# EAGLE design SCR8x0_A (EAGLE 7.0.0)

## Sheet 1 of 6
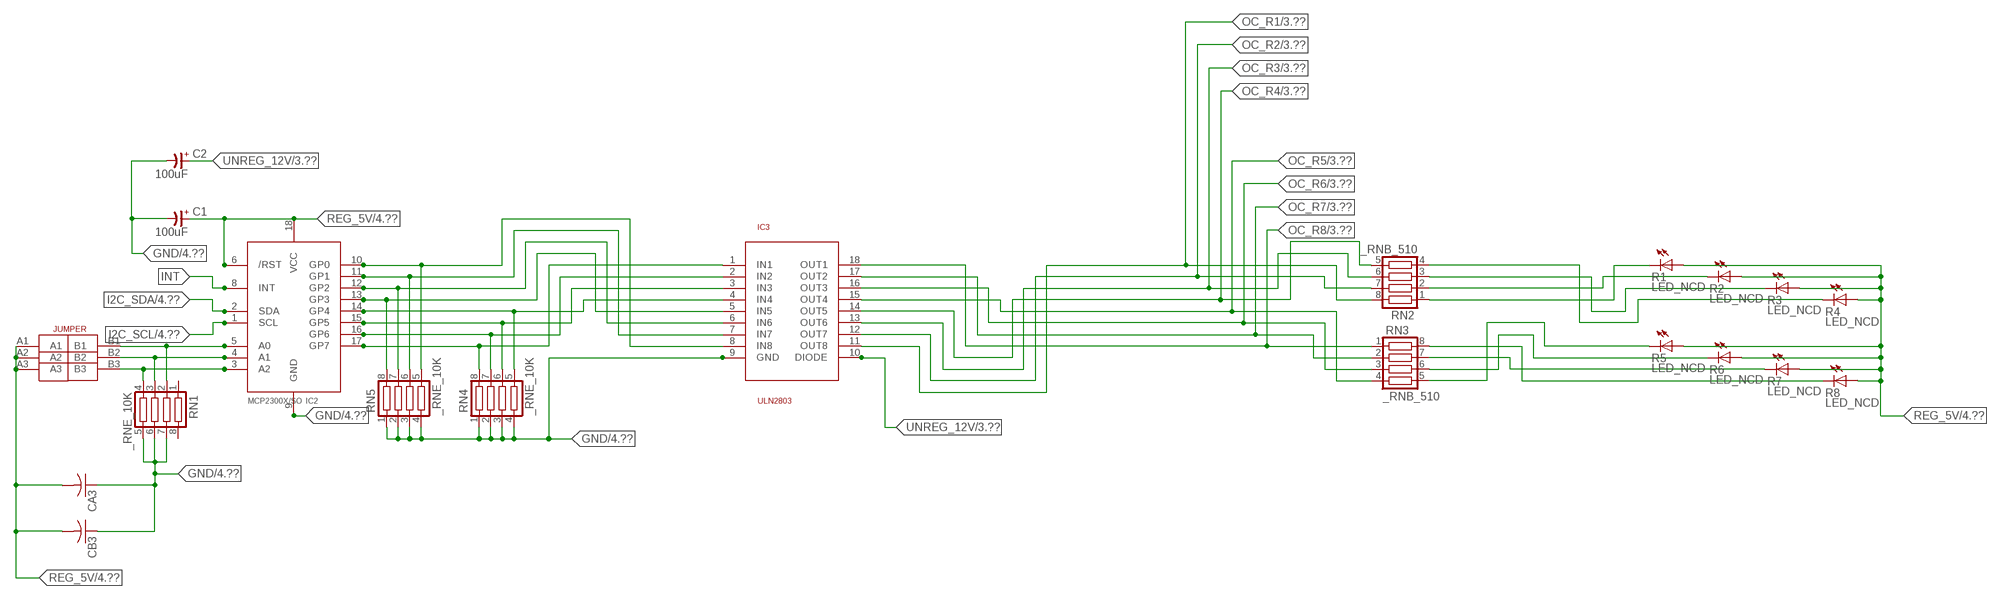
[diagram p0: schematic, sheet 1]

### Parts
C1  100uF  CP-E-025X060  [E-025X060]
C2  100uF  CP-E-025X060  [E-025X060]
CA3  CC1206KRX7R9BB104C1206K  [CC1206KRX7R9BB104]
CB3  TMK316F106ZL-TC1206K  [TMK316F106ZL-T]
IC2  MCP2300X/SO  [SO18W]
IC3  ULN2803  [SO18L]
R1  LED_NCD  [CHIPLED_0603]
R2  LED_NCD  [CHIPLED_0603]
R3  LED_NCD  [CHIPLED_0603]
R4  LED_NCD  [CHIPLED_0603]
R5  LED_NCD  [CHIPLED_0603]
R6  LED_NCD  [CHIPLED_0603]
R7  LED_NCD  [CHIPLED_0603]
R8  LED_NCD  [CHIPLED_0603]
RN1  _RNE_10K  [RNE]
RN2  _RNB_510  [RNB]
RN3  _RNB_510  [RNB]
RN4  _RNE_10K  [RNE]
RN5  _RNE_10K  [RNE]
U$18  JUMPER_3X2  [JUMPER_3X2]

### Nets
GND: C1.- C2.- CA3.1 CB3.1 IC2.9(GND) IC3.9(GND) RN1.5 RN1.6 RN1.7 RN4.1 RN4.2 RN4.3 RN4.4 RN5.1 RN5.2 RN5.3 RN5.4 ; also sheet 4,6
GP4: IC2.14(GP4) IC3.4(IN4) RN4.5
GP6: IC2.16(GP6) IC3.2(IN2) RN4.7
I2C_SCL: IC2.1(SCL) ; also sheet 4
I2C_SDA: IC2.2(SDA) ; also sheet 4
INT: IC2.8(INT)
N$6: IC2.5(A0) RN1.2 U$18.B1
N$7: IC2.4(A1) RN1.3 U$18.B2
N$8: IC2.3(A2) RN1.4 U$18.B3
N$20: R1.C RN2.1
N$21: IC2.12(GP2) IC3.6(IN6) RN5.7
N$22: IC2.11(GP1) IC3.7(IN7) RN5.6
N$23: IC2.10(GP0) IC3.8(IN8) RN5.5
N$29: R2.C RN2.2
N$30: R3.C RN2.3
N$31: R4.C RN2.4
N$32: R8.C RN3.8
N$81: R7.C RN3.7
N$82: R6.C RN3.6
N$83: R5.C RN3.5
N$89: IC2.13(GP3) IC3.5(IN5) RN5.8
N$93: IC2.15(GP5) IC3.3(IN3) RN4.6
N$94: IC2.17(GP7) IC3.1(IN1) RN4.8
OC_R1: IC3.11(OUT8) RN2.8 ; also sheet 3
OC_R2: IC3.12(OUT7) RN2.7 ; also sheet 3
OC_R3: IC3.13(OUT6) RN2.6 ; also sheet 3
OC_R4: IC3.14(OUT5) RN2.5 ; also sheet 3
OC_R5: IC3.15(OUT4) RN3.4 ; also sheet 3
OC_R6: IC3.16(OUT3) RN3.3 ; also sheet 3
OC_R7: IC3.17(OUT2) RN3.2 ; also sheet 3
OC_R8: IC3.18(OUT1) RN3.1 ; also sheet 3
REG_5V: C1.+ CA3.2 CB3.2 IC2.6(/RST) IC2.18(VCC) R1.A R2.A R3.A R4.A R5.A R6.A R7.A R8.A U$18.A1 U$18.A2 U$18.A3 ; also sheet 4,6
UNREG_12V: C2.+ IC3.10(DIODE) ; also sheet 3,4
Unconnected: RN1.1 RN1.8

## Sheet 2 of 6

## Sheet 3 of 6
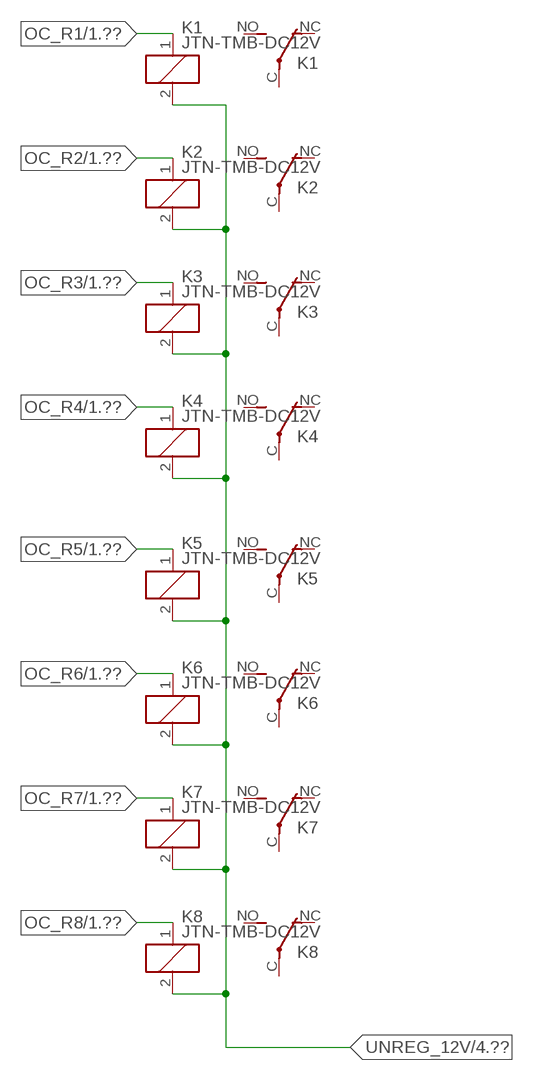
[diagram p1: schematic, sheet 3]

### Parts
K1  JTN-TMB-DC12V  [JT-TMB]
K2  JTN-TMB-DC12V  [JT-TMB]
K3  JTN-TMB-DC12V  [JT-TMB]
K4  JTN-TMB-DC12V  [JT-TMB]
K5  JTN-TMB-DC12V  [JT-TMB]
K6  JTN-TMB-DC12V  [JT-TMB]
K7  JTN-TMB-DC12V  [JT-TMB]
K8  JTN-TMB-DC12V  [JT-TMB]

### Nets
OC_R1: K1.1(C1) ; also sheet 1
OC_R2: K2.1(C1) ; also sheet 1
OC_R3: K3.1(C1) ; also sheet 1
OC_R4: K4.1(C1) ; also sheet 1
OC_R5: K5.1(C1) ; also sheet 1
OC_R6: K6.1(C1) ; also sheet 1
OC_R7: K7.1(C1) ; also sheet 1
OC_R8: K8.1(C1) ; also sheet 1
UNREG_12V: K1.2(C2) K2.2(C2) K3.2(C2) K4.2(C2) K5.2(C2) K6.2(C2) K7.2(C2) K8.2(C2) ; also sheet 1,4
Unconnected: K1.C(COM) K1.NC K1.NO K2.C(COM) K2.NC K2.NO K3.C(COM) K3.NC K3.NO K4.C(COM) K4.NC K4.NO K5.C(COM) K5.NC K5.NO K6.C(COM) K6.NC K6.NO K7.C(COM) K7.NC K7.NO K8.C(COM) K8.NC K8.NO

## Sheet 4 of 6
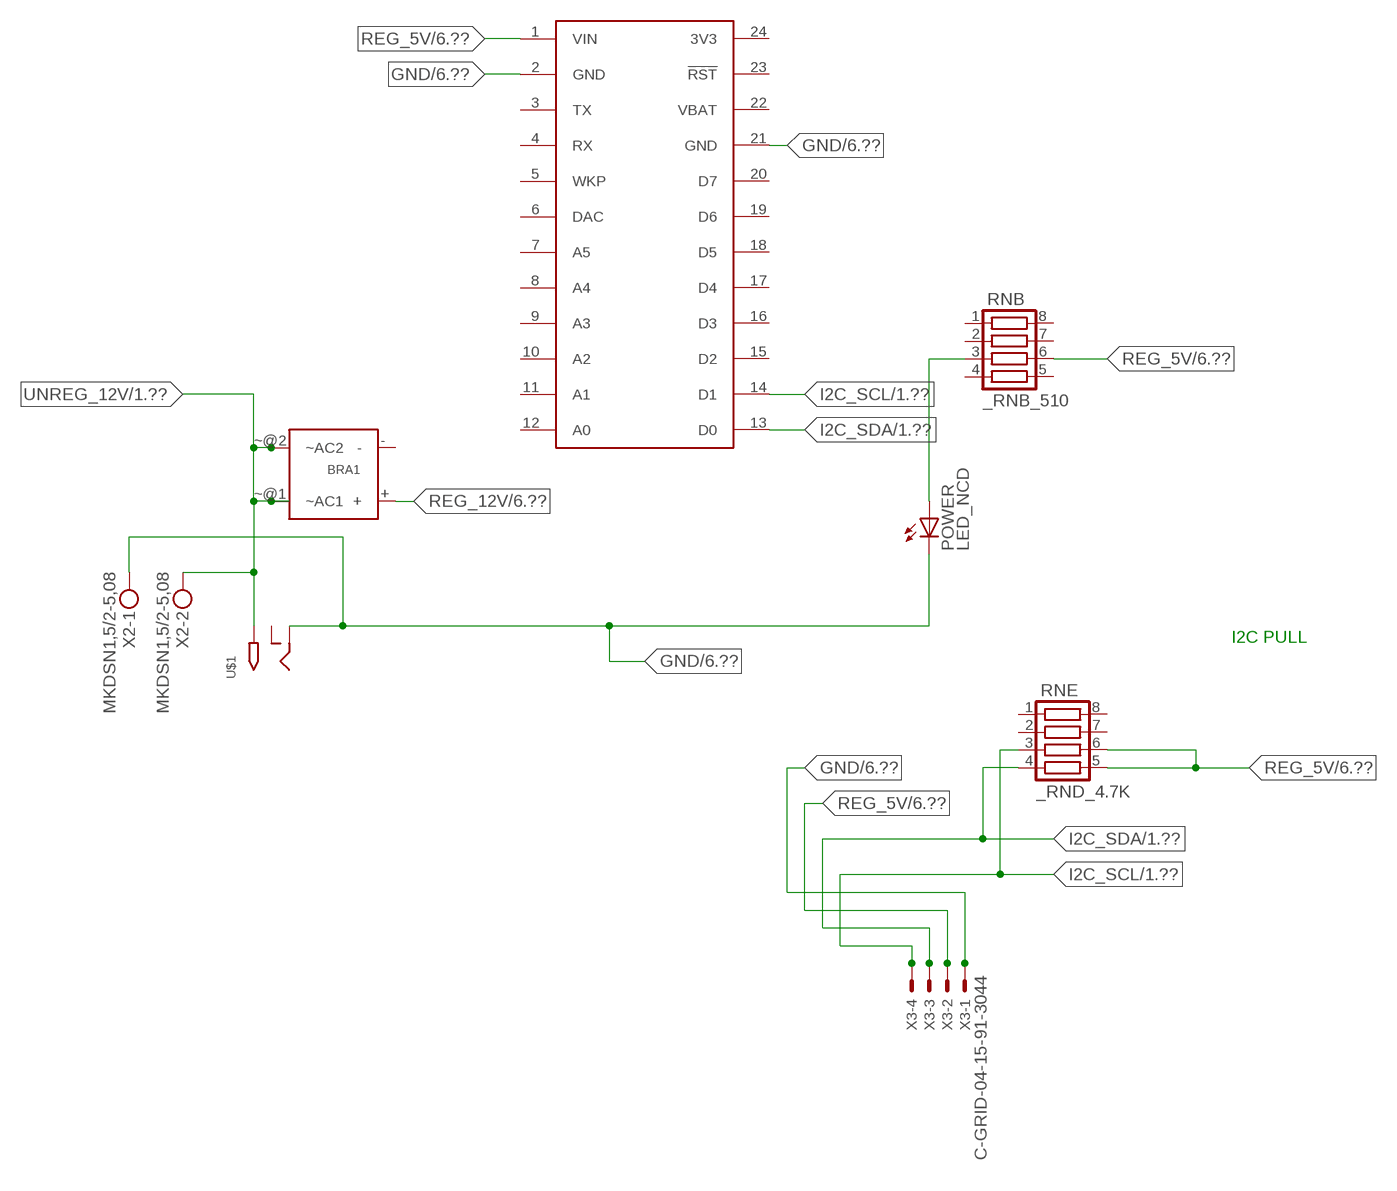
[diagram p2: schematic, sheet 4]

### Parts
BRA1  MB2S_  [MB2S]
POWER  LED_NCD  [CHIPLED_0603]
RNB  _RNB_510  [RNB]
RNE  _RND_4.7K  [RND]
S1  SPARK_CORECORE  [SPARK_CORE]
U$1  2.1MMJACK  [PJ-102A]
X2  MKDSN1,5/2-5,08  [MKDSN1,5/2-5,08]
X3  C-GRID-04-15-91-3044  [15-91-04]

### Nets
GND: POWER.C S1.2(GND) S1.21(GND) U$1.RING X2.1 X3.1 ; also sheet 1,6
I2C_SCL: RNE.3 S1.14(D1) X3.4 ; also sheet 1
I2C_SDA: RNE.4 S1.13(D0) X3.3 ; also sheet 1
N$2: POWER.A RNB.3
REG_5V: RNB.6 RNE.5 RNE.6 S1.1(VIN) X3.2 ; also sheet 1,6
REG_12V: BRA1.+ ; also sheet 6
UNREG_12V: BRA1.~@1(~AC1) BRA1.~@2(~AC2) U$1.TIP X2.2 ; also sheet 1,3
Unconnected: BRA1.- RNB.1 RNB.2 RNB.4 RNB.5 RNB.7 RNB.8 RNE.1 RNE.2 RNE.7 RNE.8 S1.3(TX) S1.4(RX) S1.5(WKP) S1.6(DAC) S1.7(A5) S1.8(A4) S1.9(A3) S1.10(A2) S1.11(A1) S1.12(A0) S1.15(D2) S1.16(D3) S1.17(D4) S1.18(D5) S1.19(D6) S1.20(D7) S1.23(!RST) U$1.RING_SW

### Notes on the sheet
- I2C PULL

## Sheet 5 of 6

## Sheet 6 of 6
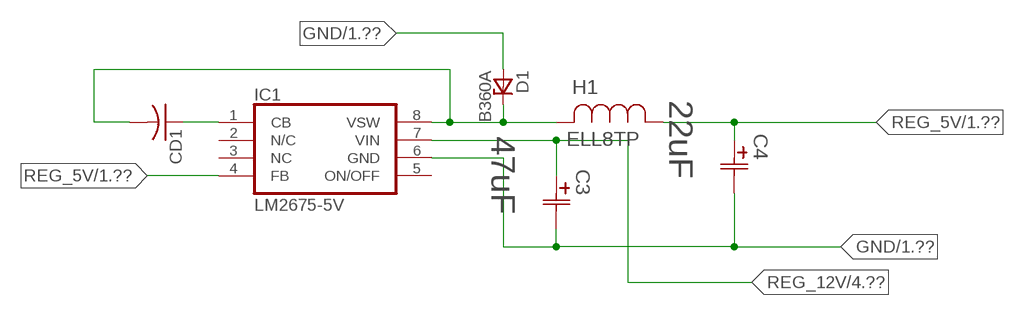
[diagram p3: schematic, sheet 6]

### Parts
C3  47uF  490-5463-6-NDCAP  [C2917(7343)-Y]
C4  22uF  490-5463-6-NDCAP  [C2917(7343)-Y]
CD1  _CD_10NF_50VC1206K  [_CD_10NF_50V]
D1  B360A  [DO214AC_ZENER]
H1  ELL8TP  [IND_ELL8TP]
IC1  LM2675-5V  LM2675  [SO-8]

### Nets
GND: C3.2(C2) C4.2(C2) D1.A IC1.6(GND) ; also sheet 1,4
N$1: CD1.2 D1.C H1.2 IC1.8(VSW)
N$3: CD1.1 IC1.1(CB)
REG_5V: C4.1(C1) H1.1 IC1.4(FB) ; also sheet 1,4
REG_12V: C3.1(C1) IC1.7(VIN) ; also sheet 4
Unconnected: IC1.2(N/C) IC1.5(ON/OFF)

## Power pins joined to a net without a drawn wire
3V3: S1.24(3V3)
NC: IC1.3(NC)
VBAT: S1.22(VBAT)

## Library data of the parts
BRA1 = NCD_ULTIMATE_LIBRARY:MB2S: Bridge Rectifier BRA MB2S 200V 500ma Digikey MB2S-TPMSTR-ND/MB2S-TP
C1 C2 = NCD_ULTIMATE_LIBRARY:CP-: Capacitors All Kinds POLARIZED CAP
C3 C4 = NCD_ULTIMATE_bhaskar:490-5463-6-ND: NCD CAP
CA3 = NCD_ULTIMATE_LIBRARY:CC1206KRX7R9BB104: Capacitor CA .1uF 50V SMT C1206K CC1206KRX7R9BB104
CB3 = NCD_ULTIMATE_LIBRARY:TMK316F106ZL-T: Capacitor CB 10uF SMT 1206 TMK316F106ZL-T
CD1 = NCD_ULTIMATE_LIBRARY:_CD_10NF_50V: Capacitor 10nF SMT
D1 = NCD_ULTIMATE_bhaskar:B360A: NCD DIODE B350A/B360A
H1 = NCD_ULTIMATE_bhaskar:ELL8TP: NCD coil
IC1 = NCD_ULTIMATE_bhaskar:LM2675: LM2675 NCD http://www.ti.com/lit/ds/symlink/lm2675.pdf
IC2 = NCD_ULTIMATE_LIBRARY:MCP2300X: Semiconductor Port Expander I/O 8-Bit I2C MCP23008 Inexpensive i2c i/o expander - 8 general purpose i/o pins with optional pullups
IC3 = NCD_ULTIMATE_LIBRARY:ULN2803: Semiconductor 8 O.C. N-Channel Transistor Driver Digikey ULN2803AFWGCELTR-ND/ULN2803AFWG,C,EL
K1-K8 = NCD_ULTIMATE_LIBRARY:JT?-*: RELAY COMPACT ECONOMICAL 30 AMP. RELAY NAiS Source: http://www.mew-europe.com/.. en_ds_61212_0000.pdf
POWER = NCD_ULTIMATE_bhaskar:LED_NCD
R1-R8 = NCD_ULTIMATE_LIBRARY:LED_NCD: LED Digikey 754-1132-2-ND/APT2012SRCPRV
RN1 RN4 RN5 = NCD_ULTIMATE_LIBRARY:_RNE_10K: Resistor Array RNE SMT 10K x 4 Single Resistor Source: http://www.ctscorp.com/components/Datasheets/CTSChipArrayDs.pdf Digikey 742C083103JPTR-ND/742C083103JP; OC_FARNELL: unknown; OC_NEWARK: unknown
RN2 RN3 RNB = NCD_ULTIMATE_LIBRARY:_RNB_510: Resistor Array RNB SMT 510 x 4 Single Resistor Source: http://www.ctscorp.com/components/Datasheets/CTSChipArrayDs.pdf Digikey 742C083511JPTR-ND/ 742C083511JP; OC_FARNELL: unknown; OC_NEWARK: unknown
RNE = NCD_ULTIMATE_LIBRARY:_RND_4.7K: Resistor Array RND SMT 4.7K x 4 Single Resistor Source: http://www.ctscorp.com/components/Datasheets/CTSChipArrayDs.pdf Digikey 742C083472JPTR-ND/742C083472JP; OC_FARNELL: unknown; OC_NEWARK: unknown
S1 = Spark:SPARK_CORE
U$1 = NCD_ULTIMATE_CONNECTORS:2.1MMJACK: 2.1mm x 5.5mm DC jack with internal switch. Digikey part #PJ-102A, 4UCON part #05537 By microbuilder.eu
U$18 = NCD_ULTIMATE_CONNECTORS:JUMPER_3X2
X2 = NCD_ULTIMATE_CONNECTORS:MKDSN1,5/2-5,08: MKDSN 1,5/ 2-5,08 Printklemme
X3 = NCD_ULTIMATE_CONNECTORS:C-GRID-04: CONNECTOR 4-Pos I2C wire to board 2.54 mm (0.100") pitch header Digikey WM1342-ND/0015912045; OC_FARNELL: unknown; OC_NEWARK: unknown

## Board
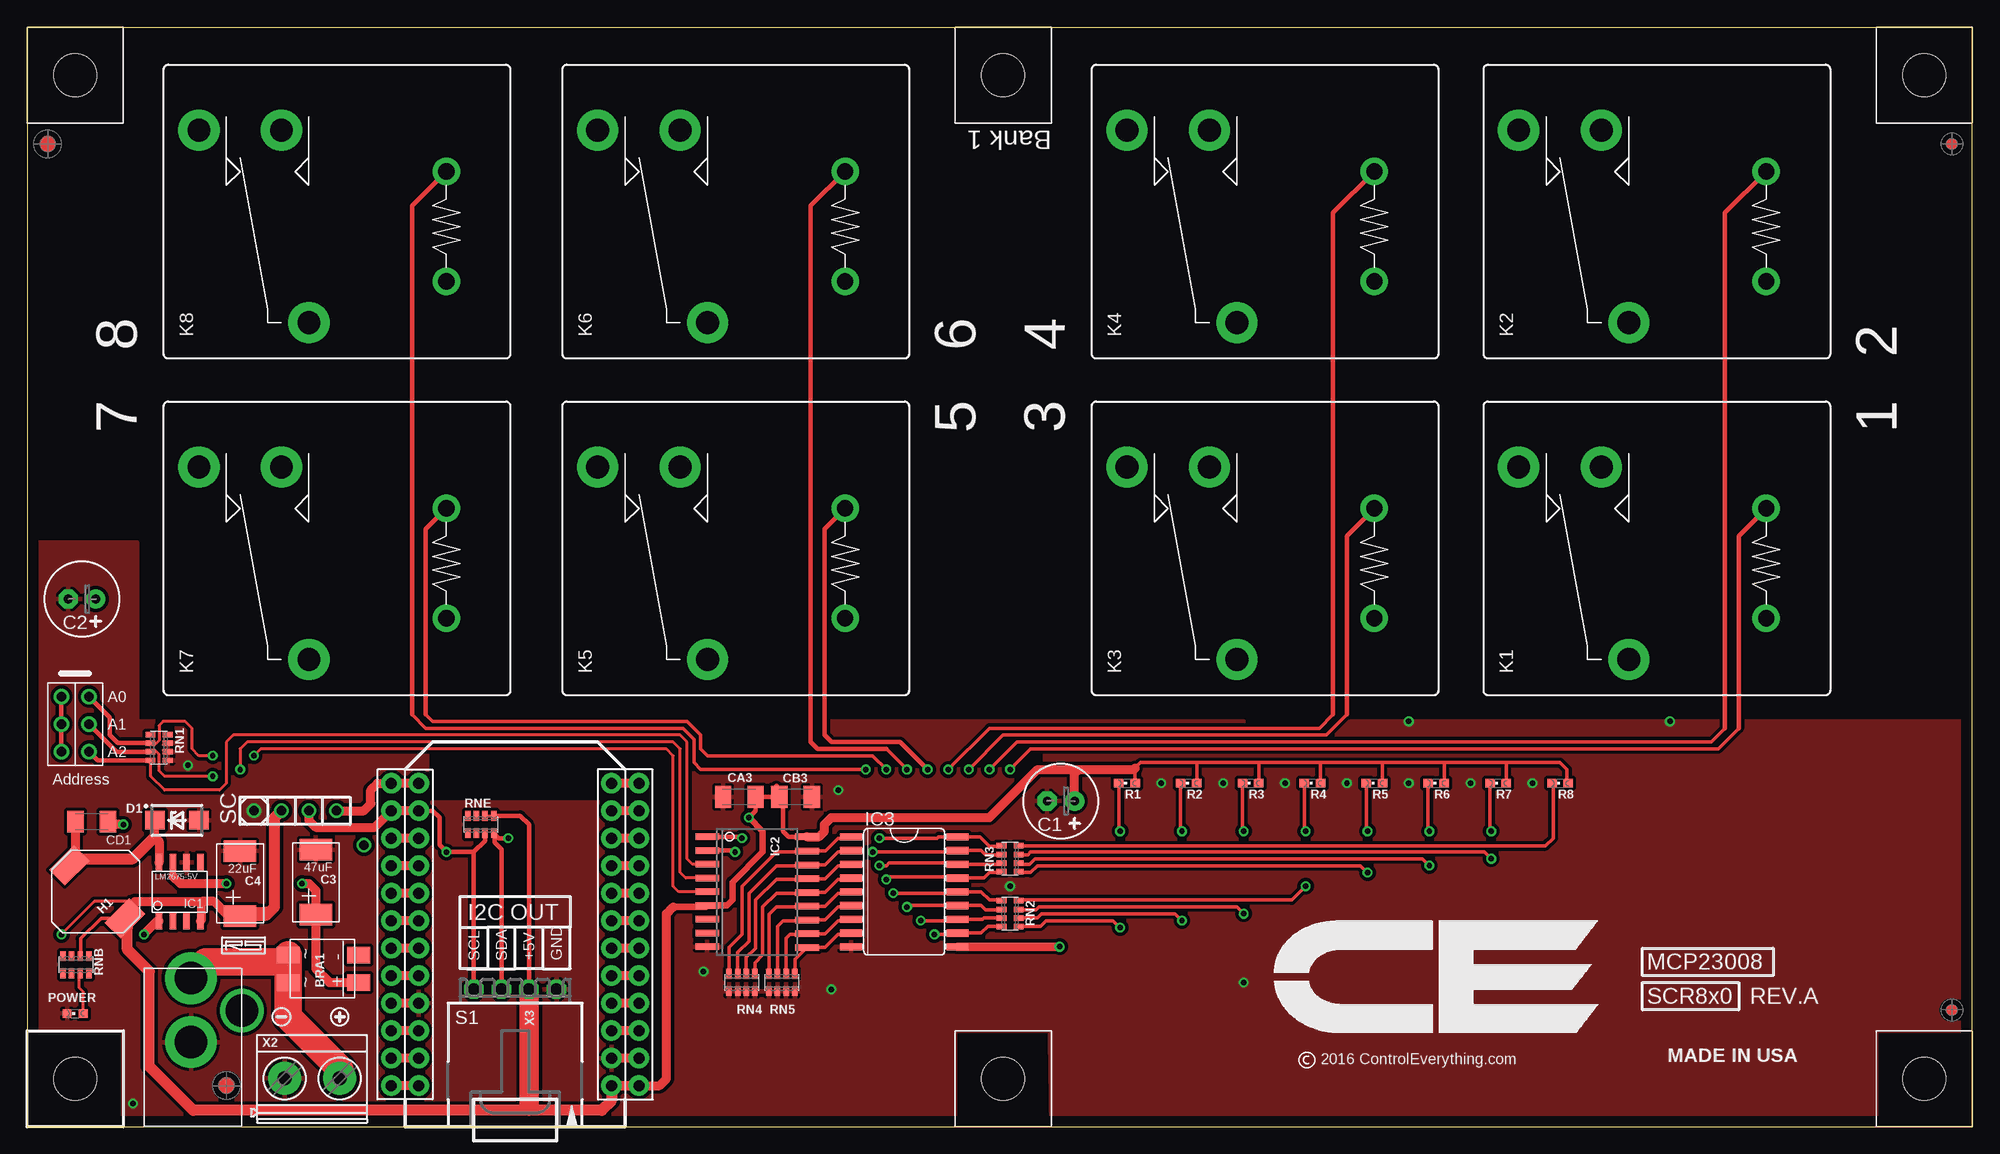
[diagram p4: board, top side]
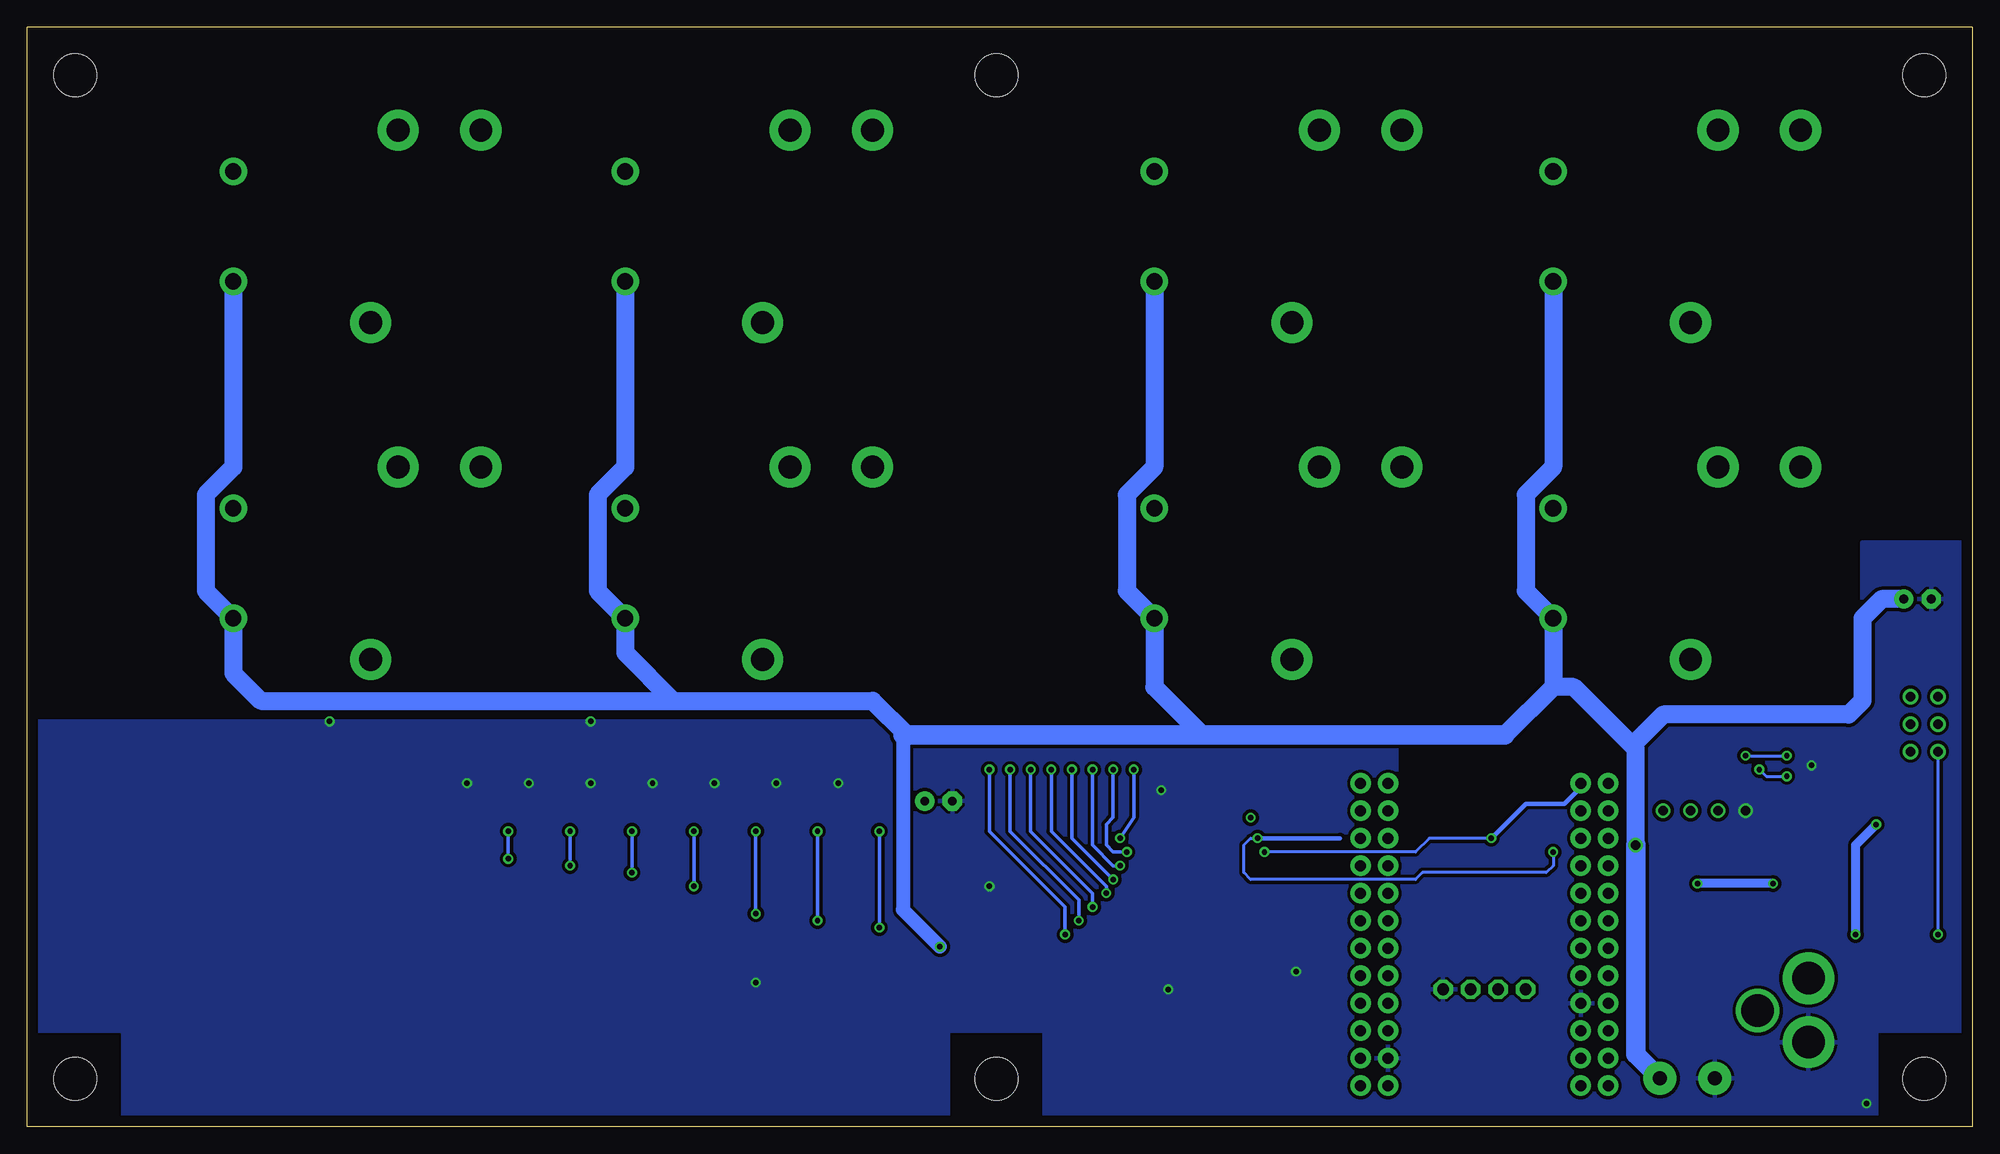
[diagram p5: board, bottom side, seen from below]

Size 179.71 x 101.61 mm. Coordinates in mm from the lower left corner, seen from the top.
Outline: 81.28,0 82.53,0
Outline: 0,59.99 0,59.05
Outline: 0,59.05 0,0 81.28,0
Outline: 81.28,0 179.71,0 179.71,101.6
Outline: 0,101.6 0,59.05
Outline: 0.02,101.61 179.71,101.61
Copper layers (1*16): Top 0.035mm / dielectric 1.5mm / Bottom 0.035mm
Design rules "default": minimum track width 10mil, minimum drill 24mil, track to track 8mil, track to pad 8mil, pad to pad 8mil, via to via 8mil, smd to smd 8mil, copper to edge 40mil, drill to drill 8mil, minimum pad ring 10mil, minimum via ring 8mil, stop-mask expansion 4mil, vias tented up to drill 0mil, thermal gap 10mil
Holes 3.96 mm at 4.45,4.45 4.45,4.45

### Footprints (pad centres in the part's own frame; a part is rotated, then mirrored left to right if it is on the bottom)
MB2S = smd 1.55 x 2.1: + 0,-6.5; - 2.54,-6.5; ~@1 0,0; ~@2 2.54,0
E-025X060 = drill 0.813 pad 1.778: + -1.27,0 | drill 0.813 pad 1.778 octagon: - 1.27,0
C2917(7343)-Y = smd 2 x 3: 1 -3,0; 2 3,0
CC1206KRX7R9BB104 = smd 1.5 x 2: 1 -1.5,0; 2 1.5,0
TMK316F106ZL-T = smd 1.5 x 2: 1 -1.5,0; 2 1.5,0
_CD_10NF_50V = smd 1.5 x 2: 1 -1.5,0; 2 1.5,0
DO214AC_ZENER = smd 1.8 x 1.7: A 2.05,0; C -2.05,0
IND_ELL8TP = smd 2.054 x 3.2 rotated 45: 1 -2.442,-2.696; 2 2.442,2.442
SO-8 = smd 0.6 x 1.55: 1 -1.905,-2.69; 2 -0.635,-2.69; 3 0.635,-2.69; 4 1.905,-2.69; 5 1.905,2.71; 6 0.635,2.71; 7 -0.635,2.71; 8 -1.905,2.71
SO18W = smd 0.6 x 2.2: 1 -4.445,-4.6; 2 -3.175,-4.6; 3 -1.905,-4.6; 4 -0.635,-4.6; 5 0.635,-4.6; 6 1.905,-4.6; 7 3.175,-4.6; 8 4.445,-4.6; 9 5.715,-4.6; 10 5.775,4.6; 11 4.505,4.6; 12 3.235,4.6; 13 1.965,4.6; 14 0.695,4.6; 15 -0.575,4.6; 16 -1.845,4.6; 17 -3.145,4.6; 18 -4.445,4.6
SO18L = smd 0.66 x 2.032: 1 -5.08,-4.902; 2 -3.81,-4.902; 3 -2.54,-4.902; 4 -1.27,-4.902; 5 0,-4.902; 6 1.27,-4.902; 7 2.54,-4.902; 8 3.81,-4.902; 9 5.08,-4.902; 10 5.08,4.902; 11 3.81,4.902; 12 2.54,4.902; 13 1.27,4.902; 14 0,4.902; 15 -1.27,4.902; 16 -2.54,4.902; 17 -3.81,4.902; 18 -5.08,4.902
JT-TMB = drill 1.5 pad 2.54: 1 5.08,0; 2 -5.08,0 | drill 2.1 pad 3.81: C -8.89,12.7; NC 8.89,22.86; NO 8.89,15.24
CHIPLED_0603 = smd 0.8 x 0.8: A 0,-0.75; C 0,0.75
CHIPLED_0603' = smd 0.8 x 0.876: A 0,-0.75; C 0,0.75
RNE = smd 0.5 x 0.9: 1 -1.2,-0.8; 2 -0.4,-0.8; 3 0.4,-0.8; 4 1.2,-0.8; 5 1.2,0.8; 6 0.4,0.8; 7 -0.4,0.8; 8 -1.2,0.8
RNB = smd 0.5 x 0.9: 1 -1.2,-0.8; 2 -0.4,-0.8; 3 0.4,-0.8; 4 1.2,-0.8; 5 1.2,0.8; 6 0.4,0.8; 7 -0.4,0.8; 8 -1.2,0.8
RND = smd 0.5 x 0.9: 1 -1.2,-0.8; 2 -0.4,-0.8; 3 0.4,-0.8; 4 1.2,-0.8; 5 1.2,0.8; 6 0.4,0.8; 7 -0.4,0.8; 8 -1.2,0.8
SPARK_CORE = drill 1.016 pad 1.88: 1 -8.89,13.97; 2 -8.89,11.43; 3 -8.89,8.89; 4 -8.89,6.35; 5 -8.89,3.81; 6 -8.89,1.27; 7 -8.89,-1.27; 8 -8.89,-3.81; 9 -8.89,-6.35; 10 -8.89,-8.89; 11 -8.89,-11.43; 12 -8.89,-13.97; 13 8.89,-13.97; 14 8.89,-11.43; 15 8.89,-8.89; 16 8.89,-6.35; 17 8.89,-3.81; 18 8.89,-1.27; 19 8.89,1.27; 20 8.89,3.81; 21 8.89,6.35; 22 8.89,8.89; 23 8.89,11.43; 24 8.89,13.97; 25 -11.43,13.97; 26 -11.43,11.43; 27 -11.43,8.89; 28 -11.43,6.35; 29 -11.43,3.81; 30 -11.43,1.27; 31 -11.43,-1.27; 32 -11.43,-3.81; 33 -11.43,-6.35; 34 -11.43,-8.89; 35 -11.43,-11.43; 36 -11.43,-13.97; 37 11.43,13.97; 38 11.43,11.43; 39 11.43,8.89; 40 11.43,6.35; 41 11.43,3.81; 42 11.43,1.27; 43 11.43,-1.27; 44 11.43,-3.81; 45 11.43,-6.35; 46 11.43,-8.89; 47 11.43,-11.43; 48 11.43,-13.97
PJ-102A = drill 3 pad 4.8: RING 0.1,-3.39; TIP 0.1,-9.29 | drill 3 pad 3.251: RING_SW -4.6,-6.29
PCB_MOUNTING_HOLE = hole 3.962: 4.445,4.445
JUMPER_3X2 = drill 0.9: A1 0,5.08; A2 0,2.54; A3 0,0; B1 2.54,5.08; B2 2.54,2.54; B3 2.54,0
MKDSN1,5/2-5,08 = drill 1.3 pad 3.048: 1 -2.561,0.025; 2 2.519,0.025
15-91-04 = drill 1.1 pad 1.778 octagon: 1 -3.81,-7.62; 2 -1.27,-7.62; 3 1.27,-7.62; 4 3.81,-7.62

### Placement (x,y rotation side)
BRA1  24.13,13.34 90 top
C1  95.5,30.1 180 top
C2  5.08,48.77 180 top
C3  26.67,22.61 90 top
C4  19.68,22.48 90 top
CA3  65.79,30.48 0 top
CB3  70.99,30.48 180 top
CD1  5.97,28.19 180 top
D1  13.84,28.32 0 top
H1  6.35,21.72 90 top
IC1  14.1,21.72 0 top
IC2  67.44,22.35 270 top
IC3  81.03,21.72 270 top
K1  160.66,52.07 90 top
K2  160.66,83.19 90 top
K3  124.46,52.07 90 top
K4  124.46,83.19 90 top
K5  75.56,52.07 90 top
K6  75.56,83.19 90 top
K7  38.73,52.07 90 top
K8  38.73,83.19 90 top
POWER  4.45,10.48 90 top
R1  LED_NCD  [CHIPLED_0603']  101.6,31.75 90 top
R2  LED_NCD  [CHIPLED_0603']  107.31,31.75 90 top
R3  LED_NCD  [CHIPLED_0603']  113.03,31.75 90 top
R4  LED_NCD  [CHIPLED_0603']  118.75,31.75 90 top
R5  LED_NCD  [CHIPLED_0603']  124.46,31.75 90 top
R6  LED_NCD  [CHIPLED_0603']  130.18,31.75 90 top
R7  LED_NCD  [CHIPLED_0603']  135.89,31.75 90 top
R8  LED_NCD  [CHIPLED_0603']  141.6,31.75 90 top
RN1  12.19,35.05 270 top
RN2  90.81,19.69 90 top
RN3  90.81,24.77 270 top
RN4  66.04,13.34 0 top
RN5  69.72,13.34 0 top
RNB  4.51,14.99 0 top
RNE  41.91,27.94 0 top
S1  45.09,17.78 180 top
U$1  15.24,4.45 180 top
U$4  [VISION_REF10]  177.8,10.79 270 top
U$6  PCB_MOUNTING_HOLE  [PCB_MOUNTING_HOLE]  94.61,0 90 top
U$10  [VISION_REF15]  18.41,3.81 0 top
U$11  PCB_MOUNTING_HOLE  [PCB_MOUNTING_HOLE]  179.71,0 90 top
U$13  [VISION_REF10]  177.8,90.8 270 top
U$14  [VISION_REF15]  1.91,90.8 270 top
U$17  PCB_MOUNTING_HOLE  [PCB_MOUNTING_HOLE]  94.61,92.71 90 top
U$18  3.17,34.67 0 top
U$19  PCB_MOUNTING_HOLE  [PCB_MOUNTING_HOLE]  94.61,92.71 90 top
U$20  PCB_MOUNTING_HOLE  [PCB_MOUNTING_HOLE]  179.71,92.71 90 top
U$21  [ICON_USA]  151.51,5.97 0 top
U$22  [ICON_MINUS]  23.5,10.16 180 top
U$24  [ICON_PLUS]  28.89,10.16 90 top
U$25  PCB_MOUNTING_HOLE  [PCB_MOUNTING_HOLE]  179.71,92.71 90 top
U$31  PCB_MOUNTING_HOLE  [PCB_MOUNTING_HOLE]  8.89,92.71 90 top
U$32  PCB_MOUNTING_HOLE  [PCB_MOUNTING_HOLE]  8.89,92.71 90 top
X2  26.35,4.45 0 top
X3  45.09,5.08 180 top

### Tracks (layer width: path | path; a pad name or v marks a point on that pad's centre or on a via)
GND  (via drill 0.5, 0.9)
  other vias: 14.86,33.4 62.48,14.35 127.64,31.75 112.39,13.34 133.35,31.75 139.06,31.75 121.92,31.75 116.2,31.75 110.49,31.75 104.78,31.75 90.81,22.23 127.64,37.46 151.76,37.46 74.3,12.7 74.93,31.12 9.78,2.16 20.95,29.21
  pour Bottom (isolate 0.305): -3.17,8.89 8.89,8.89 8.89,0 85.72,0 85.72,8.89 112.39,8.89 112.39,37.46 10.16,37.46 10.16,53.97 -3.17,53.97
  pour Top (isolate 0.305): -1.27,8.89 8.89,8.89 8.89,0 85.72,0 85.72,8.89 112.39,8.89 112.39,37.46 10.16,37.46 10.16,53.97 -1.27,53.97
  pour Top (isolate 0.305): 112.39,37.46 180.97,37.46 181.61,8.89 170.81,8.89 170.81,0 112.39,0
  pour Bottom (isolate 0.305): 94.61,0 94.61,37.46 182.25,37.46 182.88,8.89 170.81,8.89 170.81,0
  pour Top (isolate 0.305): 185.42,8.89 170.81,8.89 170.81,0 94.61,0 93.98,37.46 184.78,37.46
  pour Top (isolate 0.305): 170.81,8.89 170.81,0 94.61,0 93.98,37.46 186.69,37.46 187.32,8.89
GP4
  Top 0.305: RN4.5 67.24,15.17 67.94,15.88 67.94,20.32 69.22,21.59 71.97,21.59 IC2.14 73.73,21.66 74.93,22.86 76,22.86 IC3.4
GP6
  Top 0.305: RN4.7 65.64,16.11 66.67,17.14 66.67,21.59 69.22,24.13 71.97,24.13 IC2.16 73.73,24.2 74.93,25.4 76,25.4 IC3.2
I2C_SCL  (via drill 0.5, 0.9)
  Top 0.406: IC2.1 65.91,26.8 v66.04,26.67 | X3.4 41.27,25.4 | 41.27,25.4 42.29,26.42 42.29,27.12 RNE.3 | S1.14 37.47,29.21 38.1,28.57 38.1,26.04 v38.73,25.4 41.27,25.4
  Top 0.813: v26.04,29.21 26.04,28.32 26.67,27.69 32.13,27.69 33.66,29.21
  Bottom 0.254: v38.73,25.4 38.73,24.13 39.37,23.5 50.8,23.5 51.44,22.86 66.67,22.86 67.31,23.5 67.31,26.04 66.67,26.67 v66.04,26.67
  Bottom 0.406: v66.04,26.67 58.42,26.67
I2C_SDA  (via drill 0.5, 0.9)
  Top 0.406: IC2.2 65.28,25.53 v65.41,25.4 | X3.3 43.81,25.65 43.18,26.29 43.18,27.07 RNE.4 43.58,26.67 v44.45,26.67
  Top 0.813: v28.57,29.21 31.11,29.21 31.75,29.85 31.75,31.12 32.38,31.75 33.66,31.75
  Bottom 0.254: v44.45,26.67 50.16,26.67 51.44,25.4 v65.41,25.4
  Bottom 0.406: S1.13 36.2,31.37 37.72,29.85 41.27,29.85 v44.45,26.67
N$1
  Top 0.813: H1.2 3.88,24.77 | D1.C 11.79,26.78 12.19,26.38 IC1.8 | CD1.2 4.47,24.79 4.45,24.77
  Top 1.016: 3.88,24.77 4.45,24.77 9.78,24.77 11.79,26.78
N$2
  Top 0.254: POWER.A 5.2,12.46 4.83,12.83 4.83,14.1 RNB.3
  Top 0.406: 4.95,14.14 RNB.3
N$3  (via drill 0.5)
  Top 0.813: IC1.1 12.04,19.03 v10.79,17.78 | v8.89,27.94 7.72,27.94 CD1.1
  Bottom 0.813: v10.79,17.78 10.79,26.04 v8.89,27.94
N$6  (via drill 0.5)
  Top 0.254: IC2.5 60.2,21.72 59.69,22.23 59.69,34.29 59.05,34.92 21.59,34.92 v20.95,34.29 | v17.14,34.29 15.88,34.29 15.24,34.92 15.24,36.83 14.61,37.46 12.57,37.46 12.19,37.08 12.19,35.69 11.94,35.43 11.41,35.43 RN1.2
  Top 0.406: RN1.2 8.36,35.45 7.62,36.2 7.62,37.85 U$18.B1
  Bottom 0.254: v20.95,34.29 v17.14,34.29
N$7  (via drill 0.5)
  Top 0.254: IC2.4 60.83,22.99 60.33,23.5 60.33,34.92 59.69,35.56 20.32,35.56 19.68,34.92 v19.68,33.02 | v17.14,32.38 12.7,32.38 12.19,32.89 12.19,34.42 11.94,34.67 11.41,34.67 RN1.3
  Top 0.406: RN1.3 8.27,34.65 U$18.B2
  Bottom 0.254: v19.68,33.02 19.05,32.38 v17.14,32.38
N$8
  Top 0.254: IC2.3 61.47,24.26 60.96,24.77 60.96,35.56 60.33,36.2 19.05,36.2 18.41,35.56 18.41,31.75 17.78,31.12 12.7,31.12 11.43,32.38 11.43,33.81 RN1.4
  Top 0.406: RN1.4 6.53,33.85 U$18.B3
N$20  (via drill 0.5)
  Top 0.305: R1.C 100.85,27.42 v100.97,27.3 | v100.97,18.41 100.33,19.05 94.11,19.05 93.6,18.54 91.66,18.54 RN2.1
  Bottom 0.305: v100.97,27.3 v100.97,18.41
N$21
  Top 0.305: RN5.7 69.32,18.52 69.85,19.05 71.97,19.05 IC2.12 73.73,19.12 74.93,20.32 76,20.32 IC3.6
N$22
  Top 0.305: RN5.6 70.12,17.42 70.48,17.78 71.97,17.78 IC2.11 73.73,17.85 74.93,19.05 76,19.05 IC3.7
N$23
  Top 0.254: 71.97,16.51 IC2.10
  Top 0.305: RN5.5 70.92,15.46 IC2.10 73.73,16.58 74.93,17.78 76,17.78 IC3.8
N$29  (via drill 0.5)
  Top 0.305: R2.C 106.56,27.42 v106.68,27.3 | v106.68,19.05 106.05,19.69 93.73,19.69 93.34,19.3 91.62,19.3 RN2.2
  Bottom 0.305: v106.68,27.3 v106.68,19.05
N$30  (via drill 0.5)
  Top 0.305: R3.C 112.28,27.42 v112.39,27.3 | v112.39,19.69 111.76,20.32 93.47,20.32 93.22,20.07 91.62,20.07 RN2.3
  Bottom 0.305: v112.39,27.3 v112.39,19.69
N$31  (via drill 0.5)
  Top 0.305: R4.C 118,27.42 v118.11,27.3 | v118.11,22.23 116.84,20.96 91.67,20.96 RN2.4
  Bottom 0.305: v118.11,27.3 v118.11,22.23
N$32
  Top 0.305: RN3.8 140.26,25.96 140.97,26.67 140.97,31.64 R8.C
N$81  (via drill 0.5)
  Top 0.305: R7.C 135.14,27.42 v135.25,27.3 | v135.25,24.77 134.62,25.4 92.71,25.4 92.46,25.15 91.62,25.15 RN3.7
  Bottom 0.305: v135.25,27.3 v135.25,24.77
N$82  (via drill 0.5)
  Top 0.305: R6.C 129.43,27.42 v129.54,27.3 | v129.54,24.13 128.91,24.77 93.09,24.77 92.58,24.26 91.71,24.26 RN3.6
  Bottom 0.305: v129.54,27.3 v129.54,24.13
N$83  (via drill 0.5)
  Top 0.305: R5.C 123.71,27.42 v123.83,27.3 | v123.83,23.5 123.19,24.13 93.34,24.13 92.71,23.5 91.67,23.5 RN3.5
  Bottom 0.305: v123.83,27.3 v123.83,23.5
N$89
  Top 0.305: RN5.8 68.52,19.63 69.22,20.32 71.97,20.32 IC2.13 73.73,20.39 74.93,21.59 76,21.59 IC3.5
N$93
  Top 0.305: RN4.6 66.44,15.64 67.31,16.51 67.31,20.96 69.22,22.86 71.97,22.86 IC2.15 73.73,22.93 74.93,24.13 76,24.13 IC3.3
N$94
  Top 0.305: RN4.8 64.84,16.58 66.04,17.78 66.04,22.23 69.22,25.4 71.94,25.4 IC2.17 73.76,25.5 74.93,26.67 76,26.67 IC3.1
OC_R1  (via drill 0.5)
  Top 0.305: RN2.8 89.95,18.54 88.77,18.54 88.14,17.91 IC3.11 85.8,17.78 v83.82,17.78 | v90.81,33.02 92.71,34.92 156.21,34.92 158.12,36.83
  Top 0.406: K1.1 158.12,54.61 158.12,36.83
  Bottom 0.305: v90.81,33.02 90.81,27.3 83.82,20.32 v83.82,17.78
OC_R2  (via drill 0.5)
  Top 0.305: RN2.7 89.99,19.3 88.39,19.3 88.27,19.18 IC3.12 85.8,19.05 v82.55,19.05 | v88.9,33.02 91.44,35.56 155.57,35.56 156.84,36.83
  Top 0.406: K2.1 156.84,84.45 156.84,36.83
  Bottom 0.305: v88.9,33.02 88.9,27.3 82.55,20.96 v82.55,19.05
OC_R3  (via drill 0.5)
  Top 0.305: RN2.6 89.99,20.07 88.52,20.07 88.14,20.45 IC3.13 81.53,20.45 81.41,20.32 v81.28,20.32 | 121.92,38.1 120.02,36.2 90.17,36.2 v87,33.02
  Top 0.406: K3.1 121.92,54.61 121.92,38.1
  Bottom 0.305: v87,33.02 87,27.3 81.28,21.59 v81.28,20.32
OC_R4  (via drill 0.5)
  Top 0.305: RN2.5 89.94,20.96 88.9,20.96 88.14,21.72 IC3.14 85.8,21.59 v80.01,21.59 | 120.65,38.1 119.38,36.83 88.9,36.83 v85.09,33.02
  Top 0.406: K4.1 120.65,84.45 120.65,38.1
  Bottom 0.305: v85.09,33.02 85.09,27.3 80.01,22.23 v80.01,21.59
OC_R5  (via drill 0.5)
  Top 0.305: RN3.4 89.94,23.5 88.9,23.5 88.39,22.99 IC3.15 85.8,23.11 79.63,23.11 v79.38,22.86
  Top 0.406: K5.1 73.66,55.24 73.66,36.2 74.3,35.56 80.64,35.56 v83.19,33.02
  Bottom 0.305: v83.19,33.02 83.19,26.67 v79.38,22.86
OC_R6  (via drill 0.5)
  Top 0.305: RN3.3 89.9,24.26 IC3.16 85.8,24.38 79.63,24.38 79.38,24.13 v78.74,24.13 | 79.38,34.92 v81.28,33.02
  Top 0.406: K6.1 72.39,85.09 72.39,35.56 73.03,34.92 79.38,34.92
  Bottom 0.305: v81.28,33.02 81.28,26.04 79.38,24.13 v78.74,24.13
OC_R7  (via drill 0.5)
  Top 0.305: RN3.2 89.99,25.15 88.52,25.15 88.14,25.53 IC3.17 85.8,25.4 v78.11,25.4 | v79.38,33.02 78.11,34.29 62.87,34.29 62.23,34.92 62.23,36.2 60.96,37.46 37.47,37.46 36.83,38.1
  Top 0.406: K7.1 36.83,55.24 36.83,38.1
  Bottom 0.305: v79.38,33.02 79.38,28.57 80.01,27.94 80.01,26.04 79.38,25.4 v78.11,25.4
OC_R8  (via drill 0.5)
  Top 0.305: RN3.1 89.95,25.91 88.9,25.91 88.01,26.8 IC3.18 84.2,26.8 84.07,26.67 v78.74,26.67 | v77.47,33.02 62.23,33.02 61.59,33.66 61.59,35.81 60.58,36.83 36.83,36.83 35.56,38.1
  Top 0.406: K8.1 35.56,85.09 35.56,38.1
  Bottom 0.305: v77.47,33.02 77.47,28.57 v78.74,26.67
REG_5V  (via drill 0.5, 0.9)
  Top 0.254: RNE.6 RNE.5 | 9.96,20.83 6.22,20.83 v3.17,17.78
  Top 0.305: R1.A 102.35,33.13 102.87,33.66 107.95,33.66 | 107.95,33.66 113.67,33.66 | 113.67,33.66 119.38,33.66 | 119.38,33.66 125.09,33.66 | 125.09,33.66 130.81,33.66 | 130.81,33.66 136.53,33.66 | 136.53,33.66 141.6,33.66 142.24,33.02 142.24,31.87 R8.A | R7.A 136.64,33.54 136.53,33.66 | R6.A 130.93,33.54 130.81,33.66 | R5.A 125.21,33.54 125.09,33.66 | R4.A 119.5,33.54 119.38,33.66 | R3.A 113.78,33.54 113.67,33.66 | R2.A 108.06,33.54 107.95,33.66 | H1.1 6.83,19.28 4.95,17.4 4.95,15.83 RNB.6
  Top 0.406: U$18.A3 U$18.A2 U$18.A1 | IC2.18 70.36,26.8 69.85,27.3 69.85,30.76 CB3.2 CA3.2 67.29,29.19 v66.67,28.57 | RNE.5 45.55,28.74 46.35,27.94 X3.2
  Top 0.61: 69.22,31.39 CB3.2 | 59.69,20.32 62.71,20.32 IC2.6 64.64,20.45 65.15,20.96 65.15,22.61 67.94,25.4 67.94,27.3 v66.67,28.57
  Top 0.813: IC2.18 73.15,26.8 73.66,27.3 73.66,27.94 74.3,28.57 88.9,28.57 93.34,33.02 97.16,33.02 | 97.16,33.02 102.23,33.02 102.35,33.13 | C1.+ 96.77,32.64 97.16,33.02 | 16.13,20.83 9.96,20.83 H1.1 | 16.13,20.83 17.27,20.83 18.41,19.69 20.75,19.69 C4.1 | IC1.4 16.13,19.15 16.13,20.83 | S1.1 58.42,3.81 59.05,4.45 59.05,19.69 59.69,20.32
  Top 1.016: 46.35,2.16 46.35,1.52 | 46.35,1.52 15.37,1.52 11.3,5.59 11.3,14.35 9.27,16.38 9.27,18.41 H1.1 | 22.05,19.69 22.23,19.69 22.86,20.32 22.86,28.57 v23.5,29.21 | S1.1 53.98,2.41 53.09,1.52 46.35,1.52
  Top 1.27: 20.75,19.69 22.05,19.69
  Top 1.778: X3.2 46.35,2.16
  Bottom 0.254: v3.17,17.78 U$18.A3
REG_12V  (via drill 0.5)
  Top 0.61: IC1.7 13.46,23.16 | 14.1,22.48 14.15,22.48
  Top 0.813: v18.41,22.48 14.15,22.48 13.46,23.16 | v25.4,22.48 26.04,22.48 26.67,21.84 C3.1 26.67,14.61 27.94,13.34 BRA1.+
  Bottom 0.813: v18.41,22.48 v25.4,22.48
UNREG_12V  (via drill 0.5, 0.9)
  Top 0.762: v95.38,16.64 IC3.10
  Top 2.54: X2.2 28.87,5.42 24.13,10.16 BRA1.~@1 24.13,15.24 | 24.13,15.24 BRA1.~@2 | U$1.TIP 15.14,13.87 16.51,15.24 24.13,15.24
  Bottom 1.27: 98.81,36.2 98.81,20.07 v95.38,16.64
  Bottom 1.676: K2.2 160.66,60.96 163.19,58.42 163.19,49.53 K1.2 160.66,41.91 158.12,39.37 120.02,39.37 | K4.2 124.46,60.96 127,58.42 127,49.53 K3.2 124.46,43.81 120.02,39.37 | K6.2 75.56,60.96 78.11,58.42 78.11,49.53 K5.2 75.56,40.64 71.12,36.2 | K8.2 38.73,60.96 41.27,58.42 41.27,49.53 K7.2 38.73,40.64 | 120.02,39.37 101.6,39.37 98.42,36.2 | 38.73,40.64 43.18,36.2 | v31.11,26.04 31.11,34.92 31.43,35.24 | 31.43,35.24 36.83,40.64 38.73,40.64 | C2.+ 8.38,48.77 10.16,46.99 10.16,39.37 11.43,38.1 28.57,38.1 31.43,35.24
  Bottom 1.778: 98.81,36.2 98.42,36.2 71.12,36.2 43.18,36.2 | v31.11,26.04 31.11,6.71 X2.2

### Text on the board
tNames: Bank 1 | 8 | 6 | 4 | 2 | 7 | 5 | 3 | 1 | A0 | A1 | A2 | Address | SC | I2C OUT | SCL | SDA | +5V | GND | MCP23008 | SCR8x0 | REV.A | 2016 ControlEverything.com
